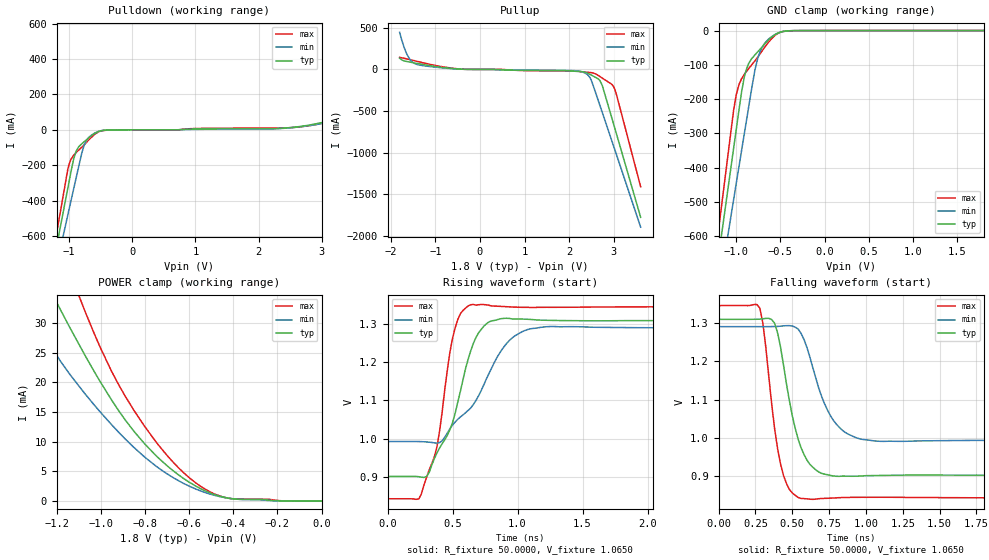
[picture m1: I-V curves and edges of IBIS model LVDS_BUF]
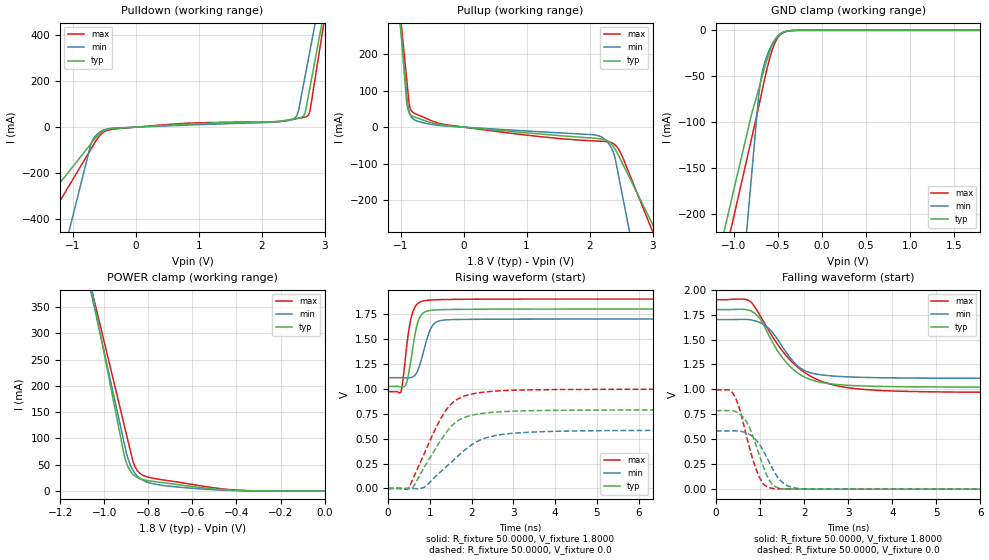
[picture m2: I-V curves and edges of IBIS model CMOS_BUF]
| TEXAS INSTRUMENTS INCORPORATED
| High Performance Analog Group
| IBIS Model for ads42lbx9 series of A/D converters
| This file provides unique models under the [Model Selector] for each
| load condition.
| For operation at a specific load condition, select the appropriate model
|after each [Model Selector] keyword.
[IBIS ver]   3.2
[File name]   ads42lbx9.ibs
[File Rev]   1.0
[Date]   Oct 24, 2012
[Source]   Data created from TI-SPICE simulations
[Disclaimer] Property of Texas Instruments Incorporated.
   Unauthorized reproduction and/or distribution is strictly
   protected under copyright law. Created 2006, (C) Copyright
   2006, Texas Instruments Incorporated, All Rights Reserved
   UNLESS THERE IS A SIGNED, WRITTEN AGREEMENT TO THE CONTRARY,
   TEXAS INSTRUMENTS (TI) IS PROVIDING THE IBIS MODELS AND
   WITHOUT ANY WARRANTY, EXPRESSED OR IMPLIED. TI assumes no
   liability for: 1) the accuracy of the IBIS models provided to
   your company; 2) the proper functioning of these IBIS Models
   in your design or for any resulting applications; or 3)
   infringement of patents, copyrights or intellectual property
   rights resulting from your use of these IBIS models. TI
   provides IBIS Models as a service to our customers. You and
   your company shall not distribute, sell or give these models
   to anyone else without prior written permission from TI.
   TI reserves the right to make changes to our products or
   to discontinue any semiconductor product or service
   without notice, and advises our customers to obtain the
   latest version of relevant information to verify, before
   placing orders, that the information being relied on is
   current.
   Please be aware that your receipt and use of the IBIS
   information provided shall serve as acceptance of these
   terms and conditions.  If you do not accept these terms,
   you should return or destroy the IBIS models and any
   other accompanying information immediately.
[Notes]   This file contains IBIS Model of various buffers of
   ads42lbx9 series of A/D converters generated with
   r_fixture of 50 ohm ( 100 ohm differential)
[Copyright]   Property of Texas Instruments Incorporated. Unauthorised
   reproduction and/or distribution is strictly prohibited. This
   product is protected under copyright law and trade secret law
   as an unpublished work. Created 2000,(C) Copyright 2000,Texas
   Instruments Inc., All Rights Reserved.These commodities are
   under the U.S. Government distribution license control.As
   such,they are not to be re-exported without the prior approval
   of the U.S. Department of Commerce.
|   Component ads42lbx9_ddr
[Component] ads42lbx9_ddr
[Manufacturer] Texas Instruments.
[Package]
| variable   typ   min   max
R_pkg   0.60837   0.52897   0.78365
L_pkg   2.09208nH   1.78421nH   2.77432nH
C_pkg   0.17978pF   0.12083pF   0.27053pF
[Pin] signal_name   model_name   R_pin   L_pin   C_pin
|   (ohms)   (nH)   (pF)
   1   DB8M   LVDS_BUF
   2   DB8P   LVDS_BUF
   3   DB6M   LVDS_BUF
   4   DB6P   LVDS_BUF
   5   DB4M   LVDS_BUF
   6   DB4P   LVDS_BUF
   7   DB2M   LVDS_BUF
   8   DB2P   LVDS_BUF
   9   DB0M   LVDS_BUF
   10   DB0P   LVDS_BUF
   11   DRVDD   POWER
|   12   CTRL2   dummy
   13   AVDD   POWER
|   14   INBP   dummy
|   15   INBM   dummy
   16   AVDD   POWER
   17   AVDD3V  POWER
|   18   SCLK   dummy
|   19   SDATA   dummy
|   20   SEN   dummy
   21   SDOUT   CMOS_BUF
|   22   RESET   dummy
   23   AVDD   POWER
|   24   CLKINM  dummy
|   25   CLKINP  dummy
   26   AVDD   POWER
|   27   VCM   dummy
|   28   RESERVED   dummy
|   29   SYNCINP dummy
|   30   SYNCINM dummy
   31   AVDD   POWER
   32   AVDD3V  POWER
   33   AVDD   POWER
|   34   INAM   dummy
|   35   INAP   dummy
   36   AVDD   POWER
|   37   CTRL1   dummy
   38   AVDD   POWER
   39   DA0M   LVDS_BUF
   40   DA0P   LVDS_BUF
   41   DA2M   LVDS_BUF
   42   DA2P   LVDS_BUF
   43   DA4M   LVDS_BUF
   44   DA4P   LVDS_BUF
   45   DA6M   LVDS_BUF
   46   DA6P   LVDS_BUF
   47   DA8M   LVDS_BUF
   48   DA8P   LVDS_BUF
   49   DRVDD   POWER
   50   DA10M   LVDS_BUF
   51   DA10P   LVDS_BUF
   52   DA12M   LVDS_BUF
   53   DA12P   LVDS_BUF
   54   DA14M   LVDS_BUF
   55   DA14P   LVDS_BUF
   56   CLKOUTM LVDS_BUF
   57   CLKOUTP LVDS_BUF
   58   DB14M   LVDS_BUF
   59   DB14P   LVDS_BUF
   60   DB12M   LVDS_BUF
   61   DB12P   LVDS_BUF
   62   DB10M   LVDS_BUF
   63   DB10P   LVDS_BUF
   64   DRVDD   POWER
[Diff Pin]   inv_pin   vdiff   tdelay_typ   tdelay_min   tdelay_max
  2   1   350mV   0   0   0
  4   3   350mV   0   0   0
  6   5   350mV   0   0   0
  8   7   350mV   0   0   0
  10   9   350mV   0   0   0
  40   39   350mV   0   0   0
  42   41   350mV   0   0   0
  44   43   350mV   0   0   0
  46   45   350mV   0   0   0
  48   47   350mV   0   0   0
  51   50   350mV   0   0   0
  53   52   350mV   0   0   0
  55   54   350mV   0   0   0
  57   56   350mV   0   0   0
  59   58   350mV   0   0   0
  61   60   350mV   0   0   0
  63   62   350mV   0   0   0
|[Series Pin Mapping]  pin_2   model_name
|   35   34   series_cap
|   14   15   series_cap
|   Component ads42lbx9_qdr
[Component] ads42lbx9_qdr
[Manufacturer] Texas Instruments.
[Package]
| variable   typ   min   max
R_pkg   0.60837   0.52897   0.78365
L_pkg   2.09208nH   1.78421nH   2.77432nH
C_pkg   0.17978pF   0.12083pF   0.27053pF
[Pin] signal_name   model_name   R_pin   L_pin   C_pin
|   (ohms)   (nH)   (pF)
1   DB1M   LVDS_BUF
2   DB1P   LVDS_BUF
3   DBCLKM  LVDS_BUF
4   DBCLKP  LVDS_BUF
5   DB2M   LVDS_BUF
6   DB2P   LVDS_BUF
7   DB3M   LVDS_BUF
8   DB3P   LVDS_BUF
9   SYNCOUTBM   LVDS_BUF
10   SYNCOUTBP   LVDS_BUF
11   DRVDD   POWER
|   12   CTRL2   dummy
13   AVDD   POWER
|   14   INBP   dummy
|   15   INBM   dummy
16   AVDD   POWER
17   AVDD3V  POWER
|   18   SCLK   dummy
|   19   SDATA   dummy
|   20   SEN   dummy
21   SDOUT   CMOS_BUF
|   22   RESET   dummy
23   AVDD   POWER
|   24   CLKP   dummy
|   25   CLKM   dummy
26   AVDD   POWER
|   27   VCM   dummy
|   28   RESV   dummy
|   29   SYNCNP  dummy
|   30   SYNCNM  dummy
31   AVDD   POWER
32   AVDD3V  POWER
33   AVDD   POWER
|   34   INAM   dummy
|   35   INAP   dummy
36   AVDD   POWER
|   37   CTRL1   dummy
38   DRVDD   POWER
39   DASTATUSM   LVDS_BUF
40   DASTATUSP   LVDS_BUF
41   DA0M   LVDS_BUF
42   DA0P   LVDS_BUF
43   DA1M   LVDS_BUF
44   DA1P   LVDS_BUF
45   DACLKM  LVDS_BUF
46   DACLKP  LVDS_BUF
47   DA2M   LVDS_BUF
48   DA2P   LVDS_BUF
49   DRVDD   POWER
50   DA3M   LVDS_BUF
51   DA3P   LVDS_BUF
52   SYNCOUTAM   LVDS_BUF
53   SYNCOUTAP   LVDS_BUF
54   OVRA   CMOS_BUF
|   55   NC   dummy
|   56   NC   dummy
|   57   NC   dummy
|   58   NC   dummy
59   OVRB   CMOS_BUF
60   DBSTATUSM   LVDS_BUF
61   DBSTATUSP   LVDS_BUF
62   DB0M   LVDS_BUF
63   DB0P   LVDS_BUF
64   DRVDD   POWER
[Diff Pin]   inv_pin   vdiff   tdelay_typ   tdelay_min   tdelay_max
  2   1   350mV   0   0   0
  4   3   350mV   0   0   0
  6   5   350mV   0   0   0
  8   7   350mV   0   0   0
  10   9   350mV   0   0   0
  40   39   350mV   0   0   0
  42   41   350mV   0   0   0
  44   43   350mV   0   0   0
  46   45   350mV   0   0   0
  48   47   350mV   0   0   0
  51   50   350mV   0   0   0
  53   52   350mV   0   0   0
  61   60   350mV   0   0   0
  63   62   350mV   0   0   0
| Models and submodels in the file (2): LVDS_BUF (Output), CMOS_BUF (3-state)
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|[Series Pin Mapping]  pin_2   model_name
|   35   34   series_cap
|   14   15   series_cap
|   Model LVDS_BUF
[Model]  LVDS_BUF
Model_type Output
Polarity   Non-Inverting
Vmeas =  1.1V
Rref =   50.0000
Vref =   1.1V
C_comp   2.5000pF   2.2500pF   2.7500pF
[Temperature Range]   25.0000   0.1250k   -40.0000
[Voltage Range]   1.8000V   1.7000V   2.0000V
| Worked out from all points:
|   slope of the pulldown table from 0 to 0.27 V, typ, clamps not added: 2.06 kohm
|   slope of the pullup table from 0 to 0.27 V, typ, clamps not added: 19 kohm
|   GND clamp passes 1 mA (typ) near -0.42 V on its own axis
|   POWER clamp passes 1 mA (typ) near -0.48 V on its own axis
|   rising waveform, R_fixture 50.0000, V_fixture 1.0650: 20-80 % time 225ps typ, 331ps min, 140ps max; typ from 0.901 V to 1.31 V
|   falling waveform, R_fixture 50.0000, V_fixture 1.0650: 20-80 % time 128ps typ, 165ps min, 96.8ps max; typ from 1.31 V to 0.901 V
[Pulldown]
|Voltage   I(typ)   I(min)   I(max)
-1.8V     -1.771A    -1.732A    -1.811A
-1.02V    -328mA     -479.8mA   -220.8mA
-890mV    -121.6mA   -273.1mA   -129.2mA
-770mV    -70.41mA   -95.96mA   -88.16mA
-690mV    -46.15mA   -44.05mA   -57.94mA
-520mV    -7.954mA   -8.025mA   -10.02mA
2.32V     7.654mA    6.289mA    10.2mA
3.16V     51.94mA    60.18mA    51.12mA
3.33V     63.36mA    166.6mA    68.7mA
3.44V     74.63mA    326.2mA    80.01mA
3.57V     107.6mA    595.5mA    90.92mA
3.6V      123.2mA    666.3mA    93.3mA
[Pullup]
|Voltage   I(typ)   I(min)   I(max)
-1.8V     135.1mA    446.1mA    145.3mA
-1.64V    94.92mA    185mA      126.6mA
-1.54V    85.13mA    101.4mA    114.1mA
-1.42V    73.1mA     61.24mA    98.52mA
-400mV    2.455mA    2.983mA    2.858mA
2.23V     -24.89mA   -21.83mA   -24.69mA
2.46V     -57.88mA   -94.82mA   -36.63mA
2.64V     -110.9mA   -357.9mA   -68.98mA
2.74V     -193.1mA   -516.9mA   -104.7mA
2.94V     -557.8mA   -836.4mA   -173.9mA
3.02V     -705.4mA   -964.6mA   -236.4mA
3.6V      -1.778A    -1.897A    -1.41A
[GND_clamp]
|Voltage   I(typ)   I(min)   I(max)
-1.8V     -1.766A    -1.727A    -1.805A
-1.03V    -342.9mA   -492.8mA   -232mA
-1V       -287.7mA   -445mA     -186.7mA
-970mV    -232.5mA   -397.3mA   -157.9mA
-910mV    -136.7mA   -302.2mA   -128.1mA
-860mV    -96.09mA   -223.1mA   -111.1mA
-790mV    -71.3mA    -116.3mA   -88.73mA
-760mV    -62.89mA   -83.49mA   -78.39mA
-690mV    -42.57mA   -41.25mA   -52.97mA
-570mV    -13.32mA   -12.85mA   -16.19mA
-360mV    -391.4uA   -482uA     -482.9uA
1.8V      55.44nA    3.177uA    33.91pA
[POWER_clamp]
|Voltage   I(typ)   I(min)   I(max)
-1.8V     117.3mA    440.3mA    111.9mA
-1.33V    43.1mA     34.45mA    57.88mA
-1.22V    34.98mA    25.77mA    46.53mA
-1.18V    32.09mA    23.46mA    42.5mA
-1.14V    29.27mA    21.38mA    38.55mA
-1.07V    24.49mA    18.03mA    31.89mA
-950mV    17mA       12.85mA    21.82mA
-850mV    11.79mA    9.06mA     15.31mA
-700mV    5.978mA    4.609mA    7.714mA
-570mV    2.537mA    2.045mA    3.081mA
-410mV    429.4uA    431.2uA    428.5uA
0V        55.44nA    189.1nA    22.56nA
[Ramp]
| variable   typ   min   max
dV/dt_r  0.3397/94.7491p   0.1993/0.1191n   0.5041/86.5313p
dV/dt_f  0.1312/0.1295n   59.9062m/0.1224n   0.2483/0.1671n
R_load = 50.0000
[Rising Waveform]
R_fixture= 50.0000
V_fixture= 1.0650
V_fixture_min= 1.1050
V_fixture_max= 1.0450
|time   V(typ)   V(min)   V(max)
0s        901.5mV    992.6mV    843.1mV
260ps     899.6mV    992.3mV    856mV
380ps     962.8mV    988.5mV    978.6mV
480ps     1.024V     1.026V     1.227V
520ps     1.066V     1.044V     1.29V
640ps     1.23V      1.08V      1.35V
760ps     1.3V       1.156V     1.35V
940ps     1.314V     1.258V     1.344V
1.24ns    1.309V     1.293V     1.343V
20ns      1.309V     1.29V      1.345V
[Falling Waveform]
R_fixture= 50.0000
V_fixture= 1.0650
V_fixture_min= 1.1050
V_fixture_max= 1.0450
|time   V(typ)   V(min)   V(max)
0s        1.309V     1.29V      1.345V
280ps     1.309V     1.29V      1.338V
380ps     1.299V     1.29V      1.025V
420ps     1.238V     1.291V     932.5mV
480ps     1.098V     1.293V     866mV
540ps     996.8mV    1.284V     844.9mV
620ps     931mV      1.21V      840.3mV
800ps     900.1mV    1.036V     843.9mV
1.1ns     902.2mV    991.1mV    845.4mV
20ns      901.4mV    992.6mV    843mV
|   Model cmos_data_high1
[Model]   CMOS_BUF
Model_type 3-state
Polarity   Non-Inverting
Enable   Active-High
Vmeas=0.9
C_comp   2.0750pF   1.9000pF   2.2500pF
[Temperature Range]   25.0000   0.1250k   -40.0000
[Voltage Range]   1.8000V   1.7000V   1.9000V
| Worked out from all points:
|   slope of the pulldown table from 0 to 0.27 V, typ, clamps not added: 61.3 ohm
|   slope of the pullup table from 0 to 0.27 V, typ, clamps not added: 62.7 ohm
|   GND clamp passes 1 mA (typ) near -0.40 V on its own axis
|   POWER clamp passes 1 mA (typ) near -0.39 V on its own axis
|   rising waveform, R_fixture 50.0000, V_fixture 1.8000: 20-80 % time 193ps typ, 247ps min, 179ps max; typ from 1.02 V to 1.8 V
|   rising waveform, R_fixture 50.0000, V_fixture 0.0: 20-80 % time 738ps typ, 988ps min, 702ps max; typ from 0 V to 0.788 V
|   falling waveform, R_fixture 50.0000, V_fixture 1.8000: 20-80 % time 731ps typ, 609ps min, 1.02ns max; typ from 1.8 V to 1.02 V
|   falling waveform, R_fixture 50.0000, V_fixture 0.0: 20-80 % time 389ps typ, 451ps min, 372ps max; typ from 0.787 V to 0 V
[Pulldown]
|Voltage   I(typ)   I(min)   I(max)
-1.8V     -446.2mA   -1.258A    -592.4mA
-720mV    -75.2mA    -81.71mA   -99.24mA
-640mV    -47.05mA   -39.01mA   -62.92mA
-460mV    -10.5mA    -8.223mA   -14.9mA
710mV     11.19mA    7.69mA     15.22mA
2.48V     34.06mA    32.63mA    32.37mA
2.55V     37.27mA    46.71mA    36.28mA
2.58V     38.61mA    65.94mA    37.79mA
2.67V     51.08mA    191.5mA    42.12mA
2.72V     102.4mA    263.3mA    46.79mA
2.77V     175.5mA    335mA      73.69mA
3.6V      1.39A      1.526A     1.509A
[Pullup]
|Voltage   I(typ)   I(min)   I(max)
-1.8V     1.985A     1.8A       1.7A
-910mV    78.41mA    98.35mA    140.6mA
-890mV    53.38mA    64.8mA     105.5mA
-860mV    37.57mA    39.26mA    59.46mA
-780mV    27.41mA    19.76mA    37.54mA
-260mV    4.234mA    2.841mA    6.131mA
2.16V     -31.57mA   -24.52mA   -38.3mA
2.28V     -36.75mA   -39.86mA   -39.94mA
2.38V     -53.19mA   -69.91mA   -45.29mA
2.47V     -80.69mA   -141.1mA   -62.92mA
2.55V     -108.6mA   -211.4mA   -92.55mA
3.6V      -474.3mA   -1.134A    -541.5mA
[GND_clamp]
|Voltage   I(typ)   I(min)   I(max)
-1.8V     -503.4mA   -1.249A    -541.8mA
-800mV    -92.85mA   -162.4mA   -119.5mA
-720mV    -65.72mA   -75.52mA   -85.37mA
-690mV    -55.13mA   -53.43mA   -71.78mA
-670mV    -48.11mA   -43.79mA   -62.73mA
-620mV    -31.66mA   -27.43mA   -41.38mA
-560mV    -15.91mA   -14.53mA   -20.65mA
-520mV    -8.804mA   -8.629mA   -11.32mA
-470mV    -3.672mA   -3.929mA   -4.772mA
-390mV    -710.2uA   -818.1uA   -1.01mA
-280mV    -32.94uA   -54.05uA   -57.7uA
1.8V      5.757nA    95.41nA    1.717nA
[POWER_clamp]
|Voltage   I(typ)   I(min)   I(max)
-1.8V     1.973A     1.793A     1.681A
-1.09V    453.9mA    436.2mA    440.9mA
-1.05V    368.3mA    359.7mA    371.1mA
-910mV    68.83mA    92.21mA    126.6mA
-890mV    43.87mA    58.68mA    91.62mA
-870mV    31.74mA    39.51mA    56.69mA
-860mV    28.17mA    33.2mA     45.72mA
-840mV    23.7mA     24.62mA    34.17mA
-800mV    19.54mA    16.1mA     26.14mA
-490mV    3.546mA    2.034mA    5.283mA
-340mV    343.4uA    193uA      468.4uA
0V        5.757nA    -261.2nA   2.433nA
[Ramp]
| variable   typ   min   max
dV/dt_r  0.4726/0.7385n   0.3503/0.9878n   0.5970/0.7015n
dV/dt_f  0.4662/0.7302n   0.3535/0.6091n   0.5577/1.0206n
R_load = 50.0000
[Rising Waveform]
R_fixture= 50.0000
V_fixture= 1.8000
V_fixture_min= 1.7000
V_fixture_max= 1.9000
|time   V(typ)   V(min)   V(max)
0s        1.023V     1.111V     970.8mV
300ps     1.02V      1.111V     962.9mV
420ps     1.038V     1.109V     1.326V
510ps     1.193V     1.11V      1.623V
600ps     1.432V     1.121V     1.779V
720ps     1.677V     1.193V     1.858V
900ps     1.774V     1.453V     1.885V
1.095ns   1.79V      1.649V     1.892V
1.47ns    1.795V     1.693V     1.896V
14.99ns   1.8V       1.7V       1.9V
[Rising Waveform]
R_fixture= 50.0000
V_fixture= 0.0
V_fixture_min= 0.0
V_fixture_max= 0.0
|time   V(typ)   V(min)   V(max)
0s        782nV      33.56uV    3.016nV
480ps     -3.858mV   -107.5uV   2.964mV
615ps     23.19mV    -1.49mV    114.2mV
870ps     215.3mV    13.64mV    353.2mV
1.395ns   563.7mV    218.8mV    789.6mV
1.695ns   685.2mV    334.3mV    903.2mV
2.13ns    744.8mV    470.2mV    957mV
2.775ns   770.8mV    543.7mV    981.3mV
4.11ns    783.8mV    573.9mV    992.3mV
14.99ns   787.6mV    583.9mV    995.1mV
[Falling Waveform]
R_fixture= 50.0000
V_fixture= 1.8000
V_fixture_min= 1.7000
V_fixture_max= 1.9000
|time   V(typ)   V(min)   V(max)
0s        1.8V       1.7V       1.9V
765ps     1.79V      1.699V     1.885V
990ps     1.712V     1.671V     1.748V
1.215ns   1.529V     1.604V     1.578V
1.5ns     1.322V     1.432V     1.39V
1.83ns    1.173V     1.244V     1.232V
2.34ns    1.075V     1.149V     1.091V
3ns       1.041V     1.125V     1.017V
5.265ns   1.025V     1.112V     973.9mV
14.99ns   1.023V     1.111V     970.4mV
[Falling Waveform]
R_fixture= 50.0000
V_fixture= 0.0
V_fixture_min= 0.0
V_fixture_max= 0.0
|time   V(typ)   V(min)   V(max)
0s        787.3mV    583.9mV    994.8mV
375ps     787.1mV    584.6mV    966.4mV
510ps     762.2mV    582.8mV    837.8mV
645ps     705.7mV    570.6mV    616.9mV
975ps     351.5mV    455.4mV    129.6mV
1.11ns    185.8mV    354.4mV    37.98mV
1.275ns   51.3mV     212.9mV    8.316mV
1.56ns    4.383mV    50.37mV    2.395mV
2.01ns    1.43mV     3.204mV    831.8uV
14.99ns   707.7nV    33.57uV    -31.28nV
